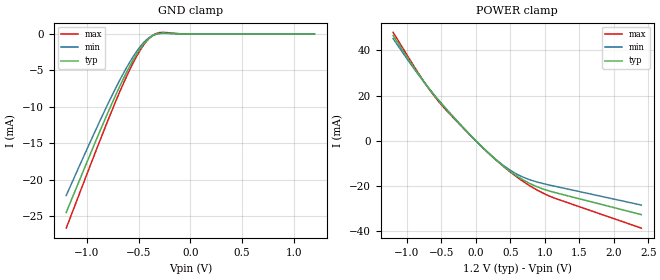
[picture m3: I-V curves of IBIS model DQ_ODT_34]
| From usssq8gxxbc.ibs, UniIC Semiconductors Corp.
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|   Model DQ_ODT_34
[Model] DQ_ODT_34
Model_type Input
Polarity   Non-Inverting
Enable   Active-High
Vinl =  8.300E-01
Vinh =  9.700E-01
C_comp   6.776E-13   6.776E-13   6.837E-13
C_comp_power_clamp   2.434E-13   2.406E-13   2.489E-13
C_comp_gnd_clamp   4.193E-13   4.187E-13   4.215E-13
[Model Spec]
Vinh   9.700E-01   9.250E-01   1.015E+00
Vinl   8.300E-01   7.850E-01   8.750E-01
[Temperature Range]   4.500E+01   9.500E+01   0.000E+00
[Voltage Range]   1.200E+00   1.140E+00   1.260E+00
[C Comp Corner]
C_comp_power_clamp   2.434E-13   2.489E-13   2.406E-13
C_comp_gnd_clamp   4.187E-13   4.193E-13   4.215E-13
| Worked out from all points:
|   GND clamp passes 1 mA (typ) near -0.43 V on its own axis
|   POWER clamp passes 1 mA (typ) near -0.03 V on its own axis
[GND_clamp]
|Voltage   I(typ)   I(min)   I(max)
-1.2V     -24.48mA   -22.16mA   -26.63mA
-850mV    -12.52mA   -11.17mA   -13.74mA
-750mV    -9.261mA   -8.22mA    -10.21mA
-650mV    -6.204mA   -5.461mA   -6.868mA
-575mV    -4.126mA   -3.597mA   -4.577mA
-500mV    -2.329mA   -2.002mA   -2.573mA
-425mV    -941.9uA   -798.6uA   -1.008mA
-375mV    -322.4uA   -281.1uA   -297.5uA
-325mV    18.72uA    -7.351uA   105uA
-275mV    127.5uA    81.46uA    229.1uA
-25mV     0A         0A         0A
1.2V      0A         0A         0A
[POWER_clamp]
|Voltage   I(typ)   I(min)   I(max)
-1.2V     46.57mA    45.23mA    47.99mA
-775mV    27.07mA    26.91mA    27.19mA
-650mV    21.95mA    22.04mA    21.71mA
-525mV    17.29mA    17.48mA    16.85mA
-225mV    7.164mA    7.214mA    6.973mA
50mV      -1.532mA   -1.526mA   -1.508mA
275mV     -8.007mA   -7.859mA   -7.982mA
475mV     -13.03mA   -12.53mA   -13.21mA
725mV     -17.98mA   -16.59mA   -18.79mA
875mV     -20.17mA   -18.11mA   -21.57mA
1.05V     -22.06mA   -19.46mA   -24.24mA
2.4V      -32.67mA   -28.44mA   -38.65mA
